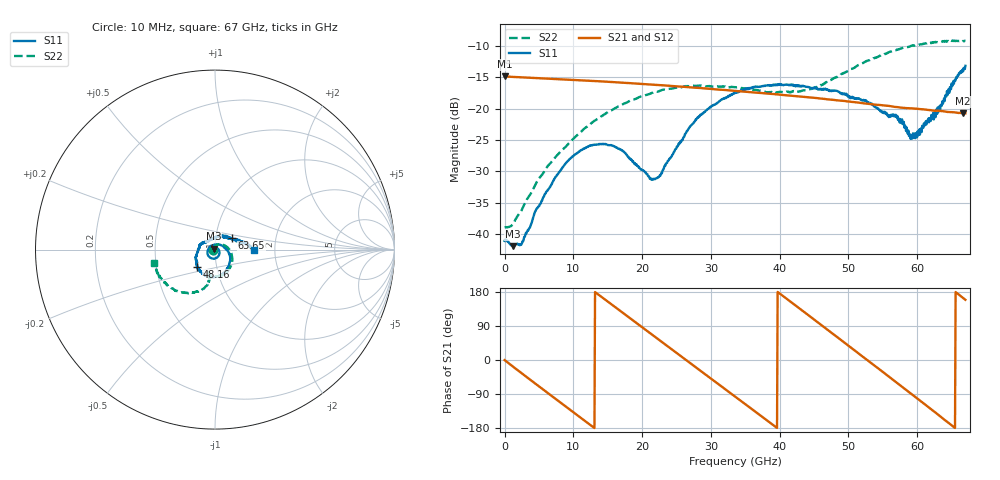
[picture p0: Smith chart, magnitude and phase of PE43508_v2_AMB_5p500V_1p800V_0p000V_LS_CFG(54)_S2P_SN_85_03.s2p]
!Keysight Technologies,N5227A,US51270237,A.10.43.00
!Date: Wednesday, August 22, 2018 17:12:13
!Correction: S11(Full 2 Port(1,3))
!S31(Full 2 Port(1,3))
!S13(Full 2 Port(1,3))
!S33(Full 2 Port(1,3))
!S2P File: Measurements: S11, S31, S13, S33:
# Hz S  dB  R 50
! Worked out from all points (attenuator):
!   801 points, 10 MHz to 67 GHz, reference 50 ohm
!   highest |S21| = -14.88 dB at 10 MHz (marker M1); lowest = -20.8 dB at 66.67 GHz (marker M2)
!   lowest |S11| = -41.9 dB at 1.182 GHz (marker M3), VSWR 1.02, Z = 49.4 + j0.532 ohm
!   |S11| at or under -10 dB: start of sweep to end of sweep
!   |S22| runs from -38.9 to -9.2 dB; largest |S21 - S12| = 0.00094
!   S11 on the Smith chart (normalised r, x): 10 MHz: 0.98, -0.00; 48.16 GHz: 0.80, -0.15; 63.65 GHz: 1.20, +0.15; 67 GHz: 1.56, -0.01
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1e7  -41.04 -177.9  -14.88 -0.2  -14.88 -0.2  -38.86 -179.3
1.182325e9  -41.87 138.1  -14.96 -16.8  -14.96 -16.8  -38.43 139.6
2.522125e9  -41.46 88.0  -15.03 -35.5  -15.03 -35.5  -36.07 107.7
6.206575e9  -33.10 -7.2  -15.22 -86.1  -15.22 -86.0  -29.27 58.7
8.886175e9  -28.70 -51.4  -15.36 -122.6  -15.36 -122.6  -26.06 34.0
1.123082e10  -26.52 -81.1  -15.50 -154.6  -15.50 -154.5  -23.58 14.3
1.566891e10  -25.87 -136.3  -15.78 145.1  -15.78 145.2  -20.21 -17.3
2.119559e10  -31.07 120.1  -16.17 70.3  -16.16 70.3  -17.60 -50.9
2.236791e10  -30.94 81.4  -16.25 54.4  -16.25 54.4  -17.25 -57.1
2.529872e10  -25.58 17.3  -16.48 14.7  -16.48 14.7  -16.61 -71.2
2.81458e10  -21.46 -17.7  -16.71 -23.8  -16.72 -23.8  -16.35 -83.5
3.3505e10  -17.52 -63.2  -17.18 -96.4  -17.18 -96.3  -16.61 -100.8
3.911541e10  -16.31 -97.3  -17.68 -172.5  -17.69 -172.3  -17.51 -106.4
4.472582e10  -16.72 -124.1  -18.24 110.6  -18.23 110.7  -16.85 -102.2
4.815906e10  -17.16 -137.0  -18.66 63.2  -18.66 63.2  -15.07 -100.7
5.201099e10  -18.70 -156.0  -19.13 9.7  -19.11 9.7  -12.82 -106.9
5.586291e10  -21.35 171.8  -19.57 -43.8  -19.57 -44.1  -11.04 -120.3
5.703524e10  -21.40 162.8  -19.76 -60.1  -19.75 -60.3  -10.62 -125.0
5.937989e10  -23.95 117.5  -19.97 -92.4  -19.99 -92.6  -9.98 -133.8
6.36505e10  -18.84 33.7  -20.40 -153.1  -20.45 -153.5  -9.34 -153.0
6.666505e10  -14.08 2.5  -20.76 163.8  -20.83 163.8  -9.25 -165.9
6.7e10  -13.20 -1.1  -20.75 158.9  -20.82 158.9  -9.24 -168.0
